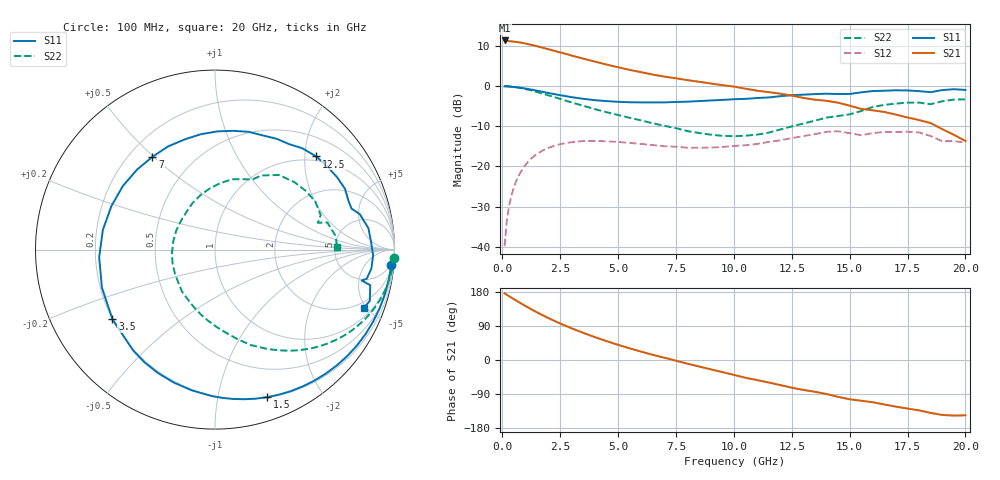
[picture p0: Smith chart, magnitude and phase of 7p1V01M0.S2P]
! Infineon Technologies  Discrete & RF Semiconductors
! bfp620
! VCE =  1.0 V,  IC =  1.0 mA
! Common Emitter S-Parameters:  Sep 2002
# GHz  S  MA  R  50
!  f  S11  S21  S12  S22
! GHz  MAG  ANG  MAG  ANG  MAG  ANG  MAG  ANG
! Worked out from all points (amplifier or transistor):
!   59 points, 100 MHz to 20 GHz, reference 50 ohm
!   highest |S21| = 11.3 dB at 100 MHz (marker M1)
!   |S21| within 3 dB of that: start of sweep to 2.521 GHz
!   unconditionally stable (mu >= 1): 6.399 GHz to 15.87 GHz; 17.6 GHz to end of sweep
!   at 1 GHz: K = 0.12, MSG = 15.1 dB, |S12| = -19.6 dB
!   at 5.5 GHz: K = 0.82, MSG = 9.1 dB, |S12| = -14.2 dB
!   at 20 GHz: K = 1.68, MAG = -4.6 dB, |S12| = -14.1 dB
!   S11 on the Smith chart (normalised r, x): 100 MHz: 3, -22; 1.5 GHz: 0.20, -1.40; 3.5 GHz: 0.20, -0.30; 7 GHz: 0.29, +0.50; 12.5 GHz: 0.90, +2.26; 20 GHz: 1.55, -4.84
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0.1  0.9866 -5.0  3.668 175.7  0.0102 85.3  0.9989 -2.8
0.2  0.9824 -9.9  3.625 172.0  0.0218 84.2  0.9949 -5.7
0.5  0.9683 -24.5  3.544 160.6  0.0548 75.3  0.9729 -13.8
1  0.9266 -48.2  3.358 142.5  0.1042 59.5  0.9135 -26.1
1.5  0.872 -70.5  3.109 125.7  0.1426 45.4  0.8386 -37.0
1.9  0.8268 -87.3  2.902 113.4  0.1653 35.4  0.7769 -44.7
2.4  0.7756 -107.1  2.651 99.0  0.1854 24.5  0.7035 -53.2
3  0.7238 -129.0  2.376 83.5  0.1997 13.0  0.6225 -62.6
3.5  0.6907 -145.8  2.181 71.5  0.2065 4.5  0.5662 -69.7
4  0.6647 -161.4  2 60.3  0.2072 -3.3  0.5135 -76.0
5  0.6343 170.1  1.703 40.0  0.2011 -15.0  0.4348 -88.1
6  0.6238 145.4  1.478 22.0  0.1901 -23.7  0.3719 -101.9
7  0.6235 124.0  1.303 6.0  0.1781 -28.9  0.3188 -117.6
8.5  0.6476 97.1  1.125 -17.2  0.1701 -32.4  0.2598 -149.6
10.5  0.69 67.1  0.923 -46.9  0.183 -36.2  0.2405 154.0
12.5  0.7668 42.6  0.758 -73.1  0.2246 -43.6  0.3136 105.2
13.5  0.7905 30.8  0.674 -83.8  0.2515 -51.7  0.3697 86.0
15  0.7943 16.7  0.568 -103.6  0.2585 -72.8  0.443 61.9
16  0.8631 7.9  0.497 -111.4  0.2591 -75.4  0.5475 49.4
17  0.8815 -2.0  0.44 -123.1  0.2677 -87.1  0.6029 32.7
18.5  0.8351 -11.9  0.345 -139.6  0.2377 -109.9  0.5923 14.6
20  0.8907 -21.3  0.207 -146.0  0.1972 -114.4  0.6814 1.4
